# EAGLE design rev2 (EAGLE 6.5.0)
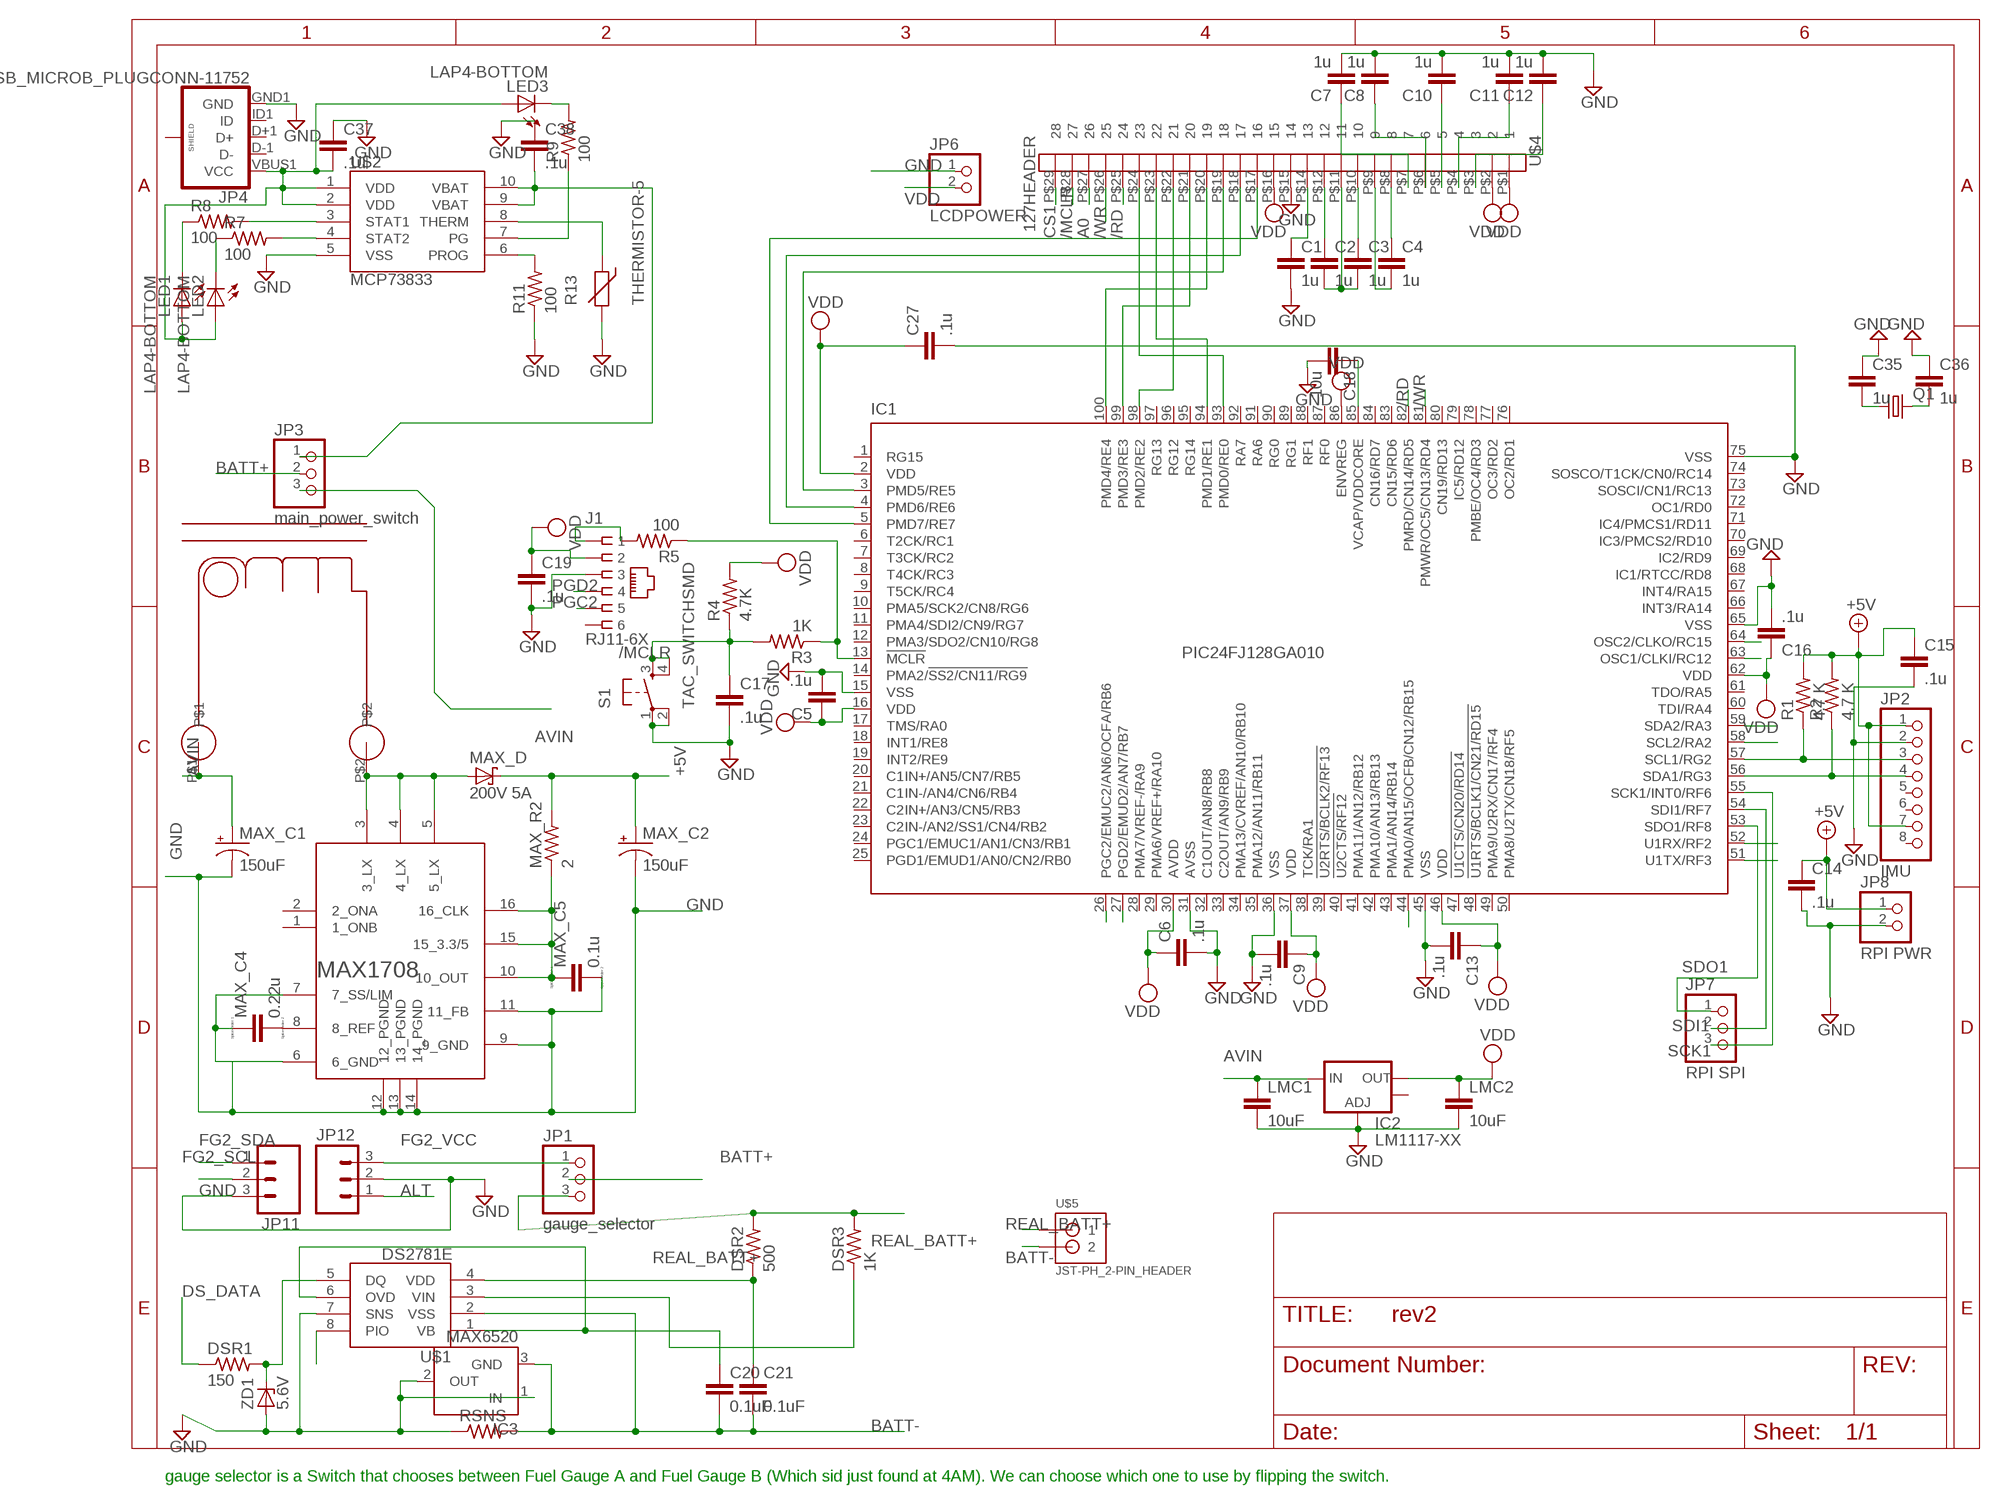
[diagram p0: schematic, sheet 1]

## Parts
C1  1u  C-EUC1206  [C1206]
C2  1u  C-EUC1206  [C1206]
C3  1u  C-EUC1206  [C1206]
C4  1u  C-EUC1206  [C1206]
C5  .1u  C-EUC1206  [C1206]
C6  .1u  C-EUC1206  [C1206]
C7  1u  C-EUC1206  [C1206]
C8  1u  C-EUC1206  [C1206]
C9  .1u  C-EUC1206  [C1206]
C10  1u  C-EUC1206  [C1206]
C11  1u  C-EUC1206  [C1206]
C12  1u  C-EUC1206  [C1206]
C13  .1u  C-EUC1206  [C1206]
C14  .1u  C-EUC1206  [C1206]
C15  .1u  C-EUC1206  [C1206]
C16  .1u  C-EUC1206  [C1206]
C17  .1u  C-EUC1206  [C1206]
C18  10u  C-EUC1206  [C1206]
C19  .1u  C-EUC1206  [C1206]
C20  0.1uF  C-EUC1206  [C1206]
C21  0.1uF  C-EUC1206  [C1206]
C27  .1u  C-EUC1206  [C1206]
C35  1u  C-EUC1206  [C1206]
C36  1u  C-EUC1206  [C1206]
C37  .1u  C-EUC1206  [C1206]
C38  .1u  C-EUC1206  [C1206]
DSR1  150  R-US_R1206  [R1206]
DSR2  500  R-US_R1206  [R1206]
DSR3  1K  R-US_R1206  [R1206]
IC1  PIC24FJ128GA010  [TQFP100-14X14]
IC2  LM1117-XX  V_REG_LM1117SOT223  [SOT223]
IC3  MAX6520  [SOT23]
J1  RJ11-6X  [RJ11-NO_SHIELD]
JP1  gauge_selector  PINHD-1X3  [1X03]
JP2  IMU  PINHD-1X8  [1X08]
JP3  main_power_switch  PINHD-1X3  [1X03]
JP4  USB_MICROB_PLUGCONN-11752  [USB-B-MICRO-SMD_V03]
JP6  LCDPOWER  PINHD-1X2  [1X02]
JP7  RPI SPI  PINHD-1X3  [1X03]
JP8  RPI PWR  PINHD-1X2  [1X02]
JP11  M03PTH  [1X03]
JP12  M03PTH  [1X03]
LED1  LAP4-BOTTOM  [P47F-BOTTOM]
LED2  LAP4-BOTTOM  [P47F-BOTTOM]
LED3  LAP4-BOTTOM  [P47F-BOTTOM]
LMC1  10uF  C-EUC1206  [C1206]
LMC2  10uF  C-EUC1206  [C1206]
MAX_C1  150uF  CPOL-USD/7343-31W  [D/7343-31W]
MAX_C2  150uF  CPOL-USD/7343-31W  [D/7343-31W]
MAX_C4  0.22u  CC1206  [C1206]
MAX_C5  0.1u  CC1206  [C1206]
MAX_D  200V 5A  SCHOTTKY-DIODESMC  [SMC]
MAX_R2  2  R-US_R1206  [R1206]
Q1  CRYTALHC49U-V  [HC49U-V]
R1  4.7 K  R-US_R1206  [R1206]
R2  4.7 K  R-US_R1206  [R1206]
R3  1K  R-US_R1206  [R1206]
R4  4.7K  R-US_R1206  [R1206]
R5  100  R-US_R1206  [R1206]
R7  100  R-US_R1206  [R1206]
R8  100  R-US_R1206  [R1206]
R9  100  R-US_R1206  [R1206]
R11  100  R-US_R1206  [R1206]
R13  THERMISTOR-5  [R-5]
RSNS  R-US_R1206  [R1206]
S1  TAC_SWITCHSMD  [TACTILE-SWITCH-SMD]
U$1  DS2781E  [TSSOP8]
U$2  MCP73833  [MSOP10]
U$3  MAX1708  [QSOP16]
U$4  127HEADER  [1.27HEADER]
U$5  JST-PH_2-PIN_HEADER  [JST_B2B-PH_HEADER]
U$6  UP2B-2R2-R  [UP2B-2R2-R]
ZD1  5.6V  ZENER-DIODESOD80C  [SOD80C]

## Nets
+5V: C14.1 C15.1 JP2.1 JP2.7 JP8.1 MAX_C2.+ MAX_D.C MAX_R2.2 R1.2 R2.2
/MCLR: C17.1 R3.2 R4.1 S1.3 S1.4 U$4.P$28
/RD: IC1.82(PMRD/CN14/RD5) U$4.P$25
/WR: IC1.81(PMWR/OC5/CN13/RD4) U$4.P$26
A0: IC1.44(PMA0/AN15/OCFB/CN12/RB15) U$4.P$27
ALT: JP12.1
AVIN: IC2.3(IN) JP3.3 LMC1.1 MAX_C1.+ U$6.P$1
BATT+: JP1.2 JP3.2
BATT-: C20.2 C21.2 IC3.3(GND) RSNS.2 U$1.2(VSS) U$5.P2
CS1: U$4.P$29
DS_DATA: DSR1.1 IC1.52(U1RX/RF2)
FG2_SCL: IC1.58(SCL2/RA2) JP11.2
FG2_SDA: IC1.59(SDA2/RA3) JP11.1
FG2_VCC: JP1.1 JP12.3
GND: C1.2 C5.2 C6.2 C7.2 C8.2 C9.2 C10.2 C11.2 C12.2 C13.2 C14.2 C15.2 C16.2 C17.2 C18.2 C19.2 C27.2 C35.1 C36.1 C37.1 C38.1 IC1.15(VSS) IC1.31(AVSS) IC1.36(VSS) IC1.45(VSS) IC1.65(VSS) IC1.75(VSS) IC2.1(ADJ) IC3.1(IN) IC3.2(OUT) J1.3 JP2.2 JP4.GND1(GND) JP6.1 JP8.2 JP11.3 JP12.2 LMC1.2 LMC2.2 MAX_C1.- MAX_C2.- MAX_C4.1 MAX_C5.2 R11.1 R13.2 RSNS.1 S1.1 S1.2 U$1.7(SNS) U$2.5(VSS) U$3.6(6_GND) U$3.7(7_SS/LIM) U$3.9(9_GND) U$3.11(11_FB) U$3.12(12_PGND) U$3.13(13_PGND) U$3.14(14_PGND) U$4.P$15 ZD1.A
N$1: IC1.57(SCL1/RG2) JP2.3 R1.1
N$2: IC1.56(SDA1/RG3) JP2.4 R2.1
N$3: LED1.C R8.1
N$4: IC1.13(!MCLR) R3.1 R5.1
N$5: R8.2 U$2.3(STAT1)
N$6: R7.2 U$2.4(STAT2)
N$7: C18.1 IC1.85(VCAP/VDDCORE)
N$8: IC1.5(PMD7/RE7) U$4.P$17
N$9: IC1.4(PMD6/RE6) U$4.P$18
N$10: IC1.3(PMD5/RE5) U$4.P$19
N$11: IC1.100(PMD4/RE4) U$4.P$20
N$12: IC1.99(PMD3/RE3) U$4.P$21
N$13: IC1.98(PMD2/RE2) U$4.P$22
N$14: IC1.94(PMD1/RE1) U$4.P$23
N$15: IC1.93(PMD0/RE0) U$4.P$24
N$16: C7.1 U$4.P$7
N$17: C3.1 U$4.P$10
N$18: LED2.C R7.1
N$19: C2.1 U$4.P$12
N$20: C2.2 C3.2 U$4.P$11
N$21: C1.1 U$4.P$14
N$22: C4.2 U$4.P$9
N$23: C4.1 U$4.P$8
N$24: C8.1 U$4.P$6
N$25: C10.1 U$4.P$5
N$26: C11.1 U$4.P$4
N$27: C12.1 U$4.P$3
N$28: R9.1 U$2.7(PG)
N$29: J1.1 R5.2
N$31: DSR1.2 U$1.5(DQ) ZD1.C
N$32: LED3.C R9.2
N$33: R11.2 U$2.6(PROG)
N$34: R13.1 U$2.8(THERM)
N$35: MAX_D.A U$3.3(3_LX) U$3.4(4_LX) U$3.5(5_LX) U$6.P$2
N$36: C21.1 DSR2.1 U$1.4(VDD)
N$37: C20.1 U$1.1(VB) U$1.6(OVD)
N$38: MAX_C5.1 MAX_R2.1 U$3.10(10_OUT) U$3.15(15_3.3/5) U$3.16(16_CLK)
N$39: DSR3.1 U$1.3(VIN)
N$40: MAX_C4.2 U$3.8(8_REF)
N$51: C38.2 JP3.1 U$2.9(VBAT) U$2.10(VBAT)
OSC1: C36.2 IC1.63(OSC1/CLKI/RC12) Q1.2
OSC2: C35.2 IC1.64(OSC2/CLKO/RC15) Q1.1
PGC2: IC1.26(PGC2/EMUC2/AN6/OCFA/RB6) J1.5
PGD2: IC1.27(PGD2/EMUD2/AN7/RB7) J1.4
PIO: IC1.51(U1TX/RF3) U$1.8(PIO)
REAL_BATT+: DSR2.2 DSR3.2 JP1.3 U$5.P1
SCK1: IC1.55(SCK1/INT0/RF6) JP7.3
SDI1: IC1.54(SDI1/RF7) JP7.2
SDO1: IC1.53(SDO1/RF8) JP7.1
VDD: C5.1 C6.1 C9.1 C13.1 C16.1 C19.1 C27.1 IC1.2(VDD) IC1.16(VDD) IC1.30(AVDD) IC1.37(VDD) IC1.46(VDD) IC1.62(VDD) IC1.86(ENVREG) IC2.2(OUT) J1.2 JP6.2 LMC2.1 R4.2 U$4.P$1 U$4.P$2 U$4.P$16
VDDUSB: C37.2 JP4.VBUS1(VCC) LED1.A LED2.A LED3.A U$2.1(VDD) U$2.2(VDD)
Unconnected: IC1.1(RG15) IC1.6(T2CK/RC1) IC1.7(T3CK/RC2) IC1.8(T4CK/RC3) IC1.9(T5CK/RC4) IC1.10(PMA5/SCK2/CN8/RG6) IC1.11(PMA4/SDI2/CN9/RG7) IC1.12(PMA3/SDO2/CN10/RG8) IC1.14(PMA2/!SS2/CN11/RG9) IC1.17(TMS/RA0) IC1.18(INT1/RE8) IC1.19(INT2/RE9) IC1.20(C1IN+/AN5/CN7/RB5) IC1.21(C1IN-/AN4/CN6/RB4) IC1.22(C2IN+/AN3/CN5/RB3) IC1.23(C2IN-/AN2/SS1/CN4/RB2) IC1.24(PGC1/EMUC1/AN1/CN3/RB1) IC1.25(PGD1/EMUD1/AN0/CN2/RB0) IC1.28(PMA7/VREF-/RA9) IC1.29(PMA6/VREF+/RA10) IC1.32(C1OUT/AN8/RB8) IC1.33(C2OUT/AN9/RB9) IC1.34(PMA13/CVREF/AN10/RB10) IC1.35(PMA12/AN11/RB11) IC1.38(TCK/RA1) IC1.39(!U2RTS/BCLK2/RF13) IC1.40(!U2CTS/RF12) IC1.41(PMA11/AN12/RB12) IC1.42(PMA10/AN13/RB13) IC1.43(PMA1/AN14/RB14) IC1.47(!U1CTS/CN20/RD14) IC1.48(!U1RTS/BCLK1/CN21/RD15) IC1.49(PMA9/U2RX/CN17/RF4) IC1.50(PMA8/U2TX/CN18/RF5) IC1.60(TDI/RA4) IC1.61(TDO/RA5) IC1.66(INT3/RA14) IC1.67(INT4/RA15) IC1.68(IC1/RTCC/RD8) IC1.69(IC2/RD9) IC1.70(IC3/PMCS2/RD10) IC1.71(IC4/PMCS1/RD11) IC1.72(OC1/RD0) IC1.73(SOSCI/CN1/RC13) IC1.74(SOSCO/T1CK/CN0/RC14) IC1.76(OC2/RD1) IC1.77(OC3/RD2) IC1.78(PMBE/OC4/RD3) IC1.79(IC5/RD12) IC1.80(CN19/RD13) IC1.83(CN15/RD6) IC1.84(CN16/RD7) IC1.87(RF0) IC1.88(RF1) IC1.89(RG1) IC1.90(RG0) IC1.91(RA6) IC1.92(RA7) IC1.95(RG14) IC1.96(RG12) IC1.97(RG13) IC2.4(OUT) J1.6 JP2.5 JP2.6 JP2.8 JP4.D+1(D+) JP4.D-1(D-) JP4.ID1(ID) JP4.SHIELD1(SHIELD) JP4.SHIELD2(SHIELD) JP4.SHIELD3(SHIELD) U$3.1(1_ONB) U$3.2(2_ONA)

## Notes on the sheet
- gauge selector is a Switch that chooses between Fuel Gauge A and Fuel Gauge B (Which sid just found at 4AM). We can choose which one to use by flipping the switch.

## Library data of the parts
C1-C21 C27 C35-C38 LMC1 LMC2 = rcl:C-EU: CAPACITOR, European symbol
DSR1-DSR3 R1-R5 R7-R9 R11 RSNS = rcl:R-US_: RESISTOR, American symbol
IC1 = microchip:PIC24FJ*GA010: 64/80/100-Pin General Purpose, 16-Bit Flash Microcontrollers Source: http://ww1.microchip.com/downloads/en/DeviceDoc/39747d.pdf; MPN: PIC24FJ128GA010-I/PT; OC_FARNELL: 1146522; OC_NEWARK: 56K7341
IC2 = SparkFun-PowerIC:V_REG_LM1117: Voltage Regulator LM1117 Standard adjustable voltage regulator but in SMD form. Spark Fun Electronics SKU : COM-00595; PROD_ID: VREG-08170
IC3 = maxim:MAX6520: 1.2V Voltage Reference 50ppm/°C, SOT23, 3-Terminal Source: Data sheet; MF: MAXIM; MPN: MAX6520EUR-T; OC_FARNELL: unknown; OC_NEWARK: 02J4586
J1 = con-tycoelectronics:RJ11: CORCOM Modular RJ Jacks No Shield Source: www.tycoelectronics.com .. ENG_DS_1654001_1099_RJ_L_0507.pdf; MPN: RJ11-6X; OC_FARNELL: unknown; OC_NEWARK: 16R6089
JP1 JP3 JP7 = pinhead:PINHD-1X3: PIN HEADER
JP2 = pinhead:PINHD-1X8: PIN HEADER
JP4 = SparkFun-Connectors:USB_MICROB_PLUG: USB Micro-B connectors Some male, some female. Watch your step!
JP6 JP8 = pinhead:PINHD-1X2: PIN HEADER
JP11 JP12 = SparkFun:M03: Header 3 Standard 3-pin 0.1" header. Use with straight break away headers (SKU : PRT-00116), right angle break away headers (PRT-00553), swiss pins (PRT-00743), machine pins (PRT-00117), and female headers (PRT-00115). Molex polarized connector foot print use with SKU : PRT-08232 with associated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
LED1-LED3 = led:*P4: PointLED® Enhanced Thinfilm LED TOP & BOTTOM mount
MAX_C1 MAX_C2 = adafruit:CPOL-US: POLARIZED CAPACITOR, American symbol
MAX_C4 MAX_C5 = eagle-ltspice:C: CAPACITOR, European symbol; SPICEMODEL: NONE; SPICEPREFIX: C
MAX_D = diode:SCHOTTKY-DIODE: Schottky Diode
MAX_R2 = adafruit:R-US_: RESISTOR, American symbol
Q1 = crystal:CRYTAL: CRYSTAL
R13 = varistor:THERMISTOR: THERMISTOR
S1 = SparkFun-Retired:TAC_SWITCH: Momentary Switch Button commonly used for reset or general input. Spark Fun Electronics SKU : COM-00097 SMT- SWCH-08247; PROD_ID: SWCH-08247
U$1 = fuelgauge:DS2781E
U$2 = fuelgauge:MCP73833
U$3 = max1708:MAX1708
U$4 = fuelgauge:127HEADER
U$5 = SRG:JST-PH_2-PIN_HEADER: 2-pin JST PH Shrouded Header, top entry
U$6 = duckgauge:UP2B-2R2-R: Yeah yeah inducktor
ZD1 = diode:ZENER-DIODE: Z-Diode

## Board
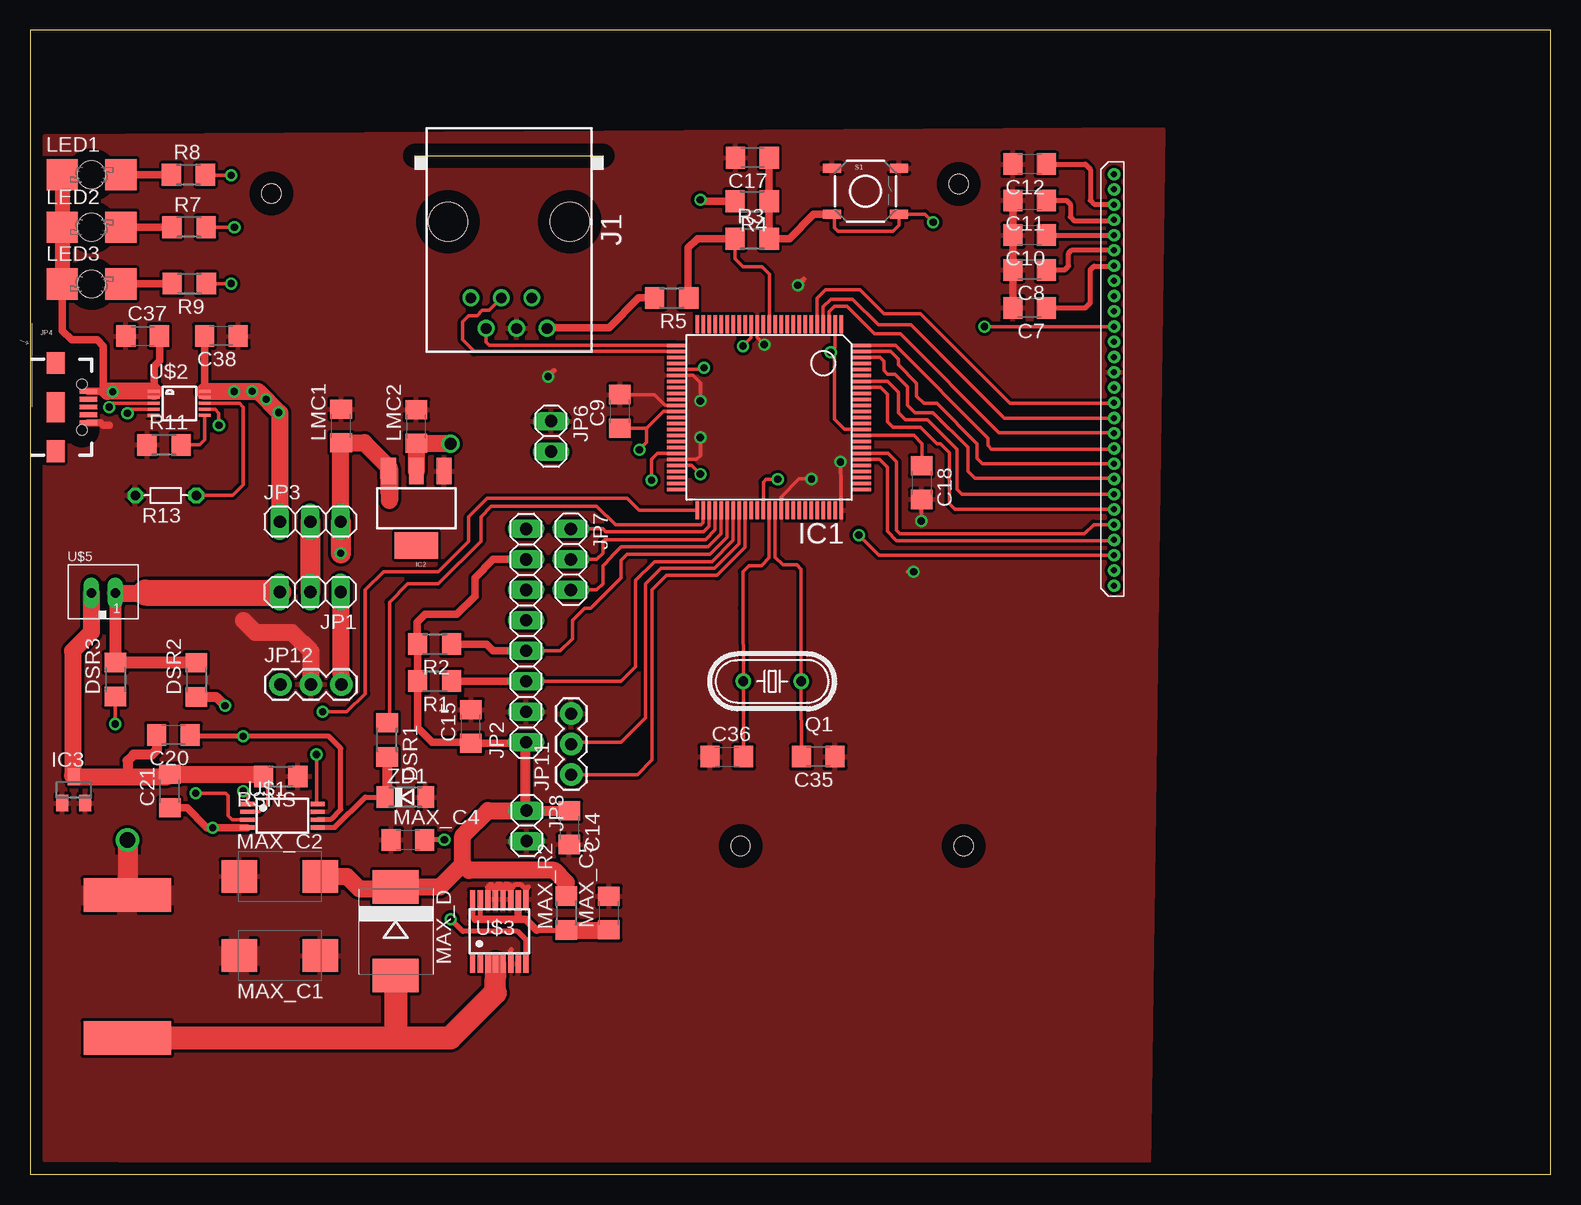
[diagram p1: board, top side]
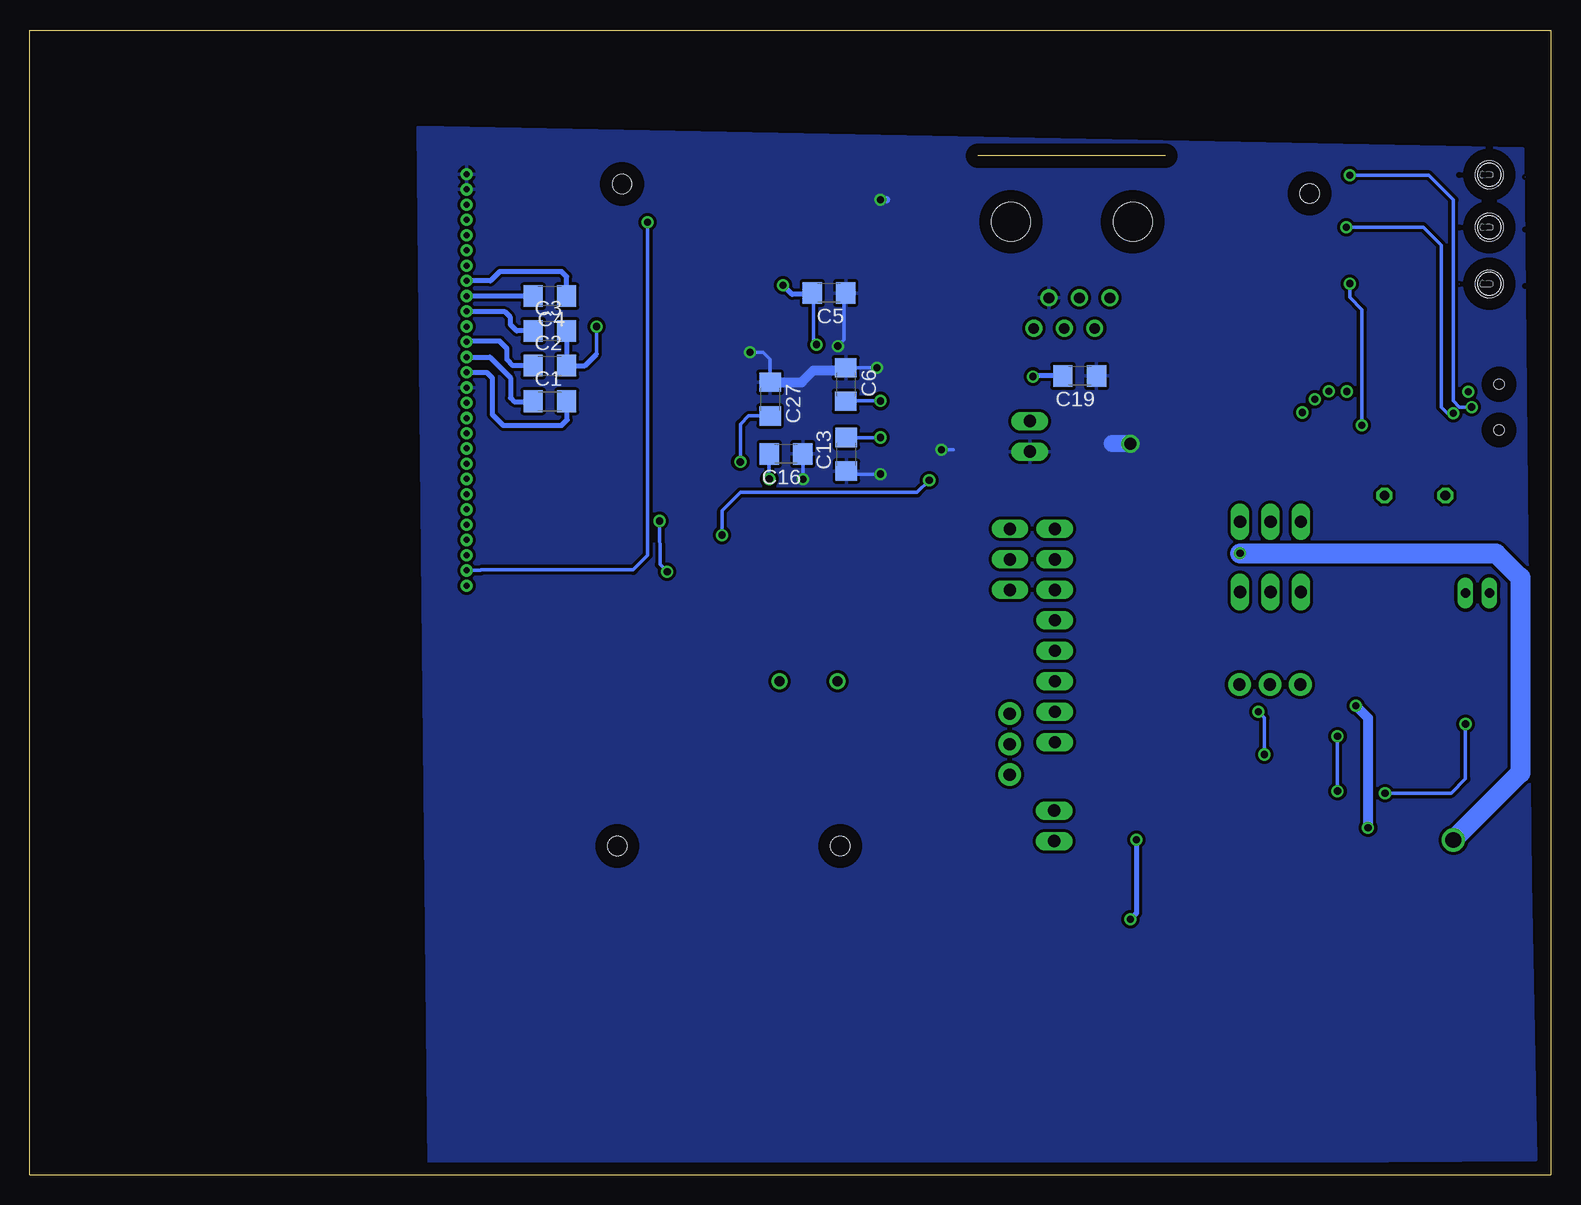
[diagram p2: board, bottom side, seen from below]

Size 126.78 x 95.4 mm. Coordinates in mm from the lower left corner, seen from the top.
Outline: 126.78,0 126.78,95.4 0,95.4 0,0 126.78,0
Copper layers (1*16): Top 0.035mm / dielectric 1.5mm / Bottom 0.035mm
Design rules "default": minimum track width 10mil, minimum drill 24mil, track to track 8mil, track to pad 8mil, pad to pad 8mil, via to via 8mil, smd to smd 8mil, copper to edge 40mil, drill to drill 8mil, minimum pad ring 10mil, minimum via ring 8mil, stop-mask expansion 4mil, vias tented up to drill 0mil, thermal gap 10mil
Holes 1.6 mm at 59.23,27.41 77.42,82.58 20.12,81.76 77.83,27.41

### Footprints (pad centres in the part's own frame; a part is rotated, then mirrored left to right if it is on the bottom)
C1206 = smd 1.6 x 1.8: 1 -1.4,0; 2 1.4,0
R1206 = smd 1.6 x 1.803: 1 -1.422,0; 2 1.422,0
TQFP100-14X14 = smd 0.27 x 1.5: 1 -6,-7.75; 2 -5.5,-7.75; 3 -5,-7.75; 4 -4.5,-7.75; 5 -4,-7.75; 6 -3.5,-7.75; 7 -3,-7.75; 8 -2.5,-7.75; 9 -2,-7.75; 10 -1.5,-7.75; 11 -1,-7.75; 12 -0.5,-7.75; 13 0,-7.75; 14 0.5,-7.75; 15 1,-7.75; 16 1.5,-7.75; 17 2,-7.75; 18 2.5,-7.75; 19 3,-7.75; 20 3.5,-7.75; 21 4,-7.75; 22 4.5,-7.75; 23 5,-7.75; 24 5.5,-7.75; 25 6,-7.75; 51 6,7.75; 52 5.5,7.75; 53 5,7.75; 54 4.5,7.75; 55 4,7.75; 56 3.5,7.75; 57 3,7.75; 58 2.5,7.75; 59 2,7.75; 60 1.5,7.75; 61 1,7.75; 62 0.5,7.75; 63 0,7.75; 64 -0.5,7.75; 65 -1,7.75; 66 -1.5,7.75; 67 -2,7.75; 68 -2.5,7.75; 69 -3,7.75; 70 -3.5,7.75; 71 -4,7.75; 72 -4.5,7.75; 73 -5,7.75; 74 -5.5,7.75; 75 -6,7.75 | smd 1.5 x 0.27: 26 7.75,-6; 27 7.75,-5.5; 28 7.75,-5; 29 7.75,-4.5; 30 7.75,-4; 31 7.75,-3.5; 32 7.75,-3; 33 7.75,-2.5; 34 7.75,-2; 35 7.75,-1.5; 36 7.75,-1; 37 7.75,-0.5; 38 7.75,0; 39 7.75,0.5; 40 7.75,1; 41 7.75,1.5; 42 7.75,2; 43 7.75,2.5; 44 7.75,3; 45 7.75,3.5; 46 7.75,4; 47 7.75,4.5; 48 7.75,5; 49 7.75,5.5; 50 7.75,6; 76 -7.75,6; 77 -7.75,5.5; 78 -7.75,5; 79 -7.75,4.5; 80 -7.75,4; 81 -7.75,3.5; 82 -7.75,3; 83 -7.75,2.5; 84 -7.75,2; 85 -7.75,1.5; 86 -7.75,1; 87 -7.75,0.5; 88 -7.75,0; 89 -7.75,-0.5; 90 -7.75,-1; 91 -7.75,-1.5; 92 -7.75,-2; 93 -7.75,-2.5; 94 -7.75,-3; 95 -7.75,-3.5; 96 -7.75,-4; 97 -7.75,-4.5; 98 -7.75,-5; 99 -7.75,-5.5; 100 -7.75,-6
SOT223 = smd 1.219 x 2.235: 1 -2.311,-3.099; 2 0,-3.099; 3 2.311,-3.099 | smd 3.6 x 2.2: 4 0,3.099
SOT23 = smd 1 x 1.4: 1 -0.95,-1.1; 2 0.95,-1.1; 3 0,1.1
RJ11-NO_SHIELD = drill 0.9 pad 1.4: 1 -3.175,8.89; 2 -1.905,6.35; 3 -0.635,8.89; 4 0.635,6.35; 5 1.905,8.89; 6 3.175,6.35 | hole 3.251: -5.08,0; 5.08,0
1X03 = drill 1.016 long: 1 -2.54,0; 2 0,0; 3 2.54,0
1X08 = drill 1.016 long: 1 -8.89,0; 2 -6.35,0; 3 -3.81,0; 4 -1.27,0; 5 1.27,0; 6 3.81,0; 7 6.35,0; 8 8.89,0
USB-B-MICRO-SMD_V03 = smd 1.45 x 0.4: D+1 2.725,0; D-1 2.725,0.65; GND1 2.725,-1.3; ID1 2.725,-0.65; VBUS1 2.725,1.3 | smd 1.5 x 1.8: SHIELD1 0,3.685; SHIELD2 0,-3.685 | smd 1.5 x 2.5: SHIELD3 0,0 | hole 0.85: 2.2,1.9; 2.2,-1.9
1X02 = drill 1.016 long: 1 -1.27,0; 2 1.27,0
1X03' = drill 1.016 pad 1.88: 1 0,0; 2 2.54,0; 3 5.08,0
P47F-BOTTOM = smd 2.6 x 2.6: A -2.45,0; C 2.45,0 | hole 2.3: 0,0
D/7343-31W = smd 2.95 x 2.7: + 3.375,0; - -3.375,0
SMC = smd 2.8 x 3.8: A 3.7,0; C -3.7,0
HC49U-V = drill 0.813: 1 -2.413,0; 2 2.413,0
R-5 = drill 0.813 octagon: 1 -2.54,0; 2 2.54,0
TACTILE-SWITCH-SMD = smd 1.524 x 0.762: 1 -2.794,1.905; 2 2.794,1.905; 3 -2.794,-1.905; 4 2.794,-1.905
TSSOP8 = smd 1.2 x 0.35: 1 -2.925,0.975; 2 -2.925,0.325; 3 -2.925,-0.325; 4 -2.925,-0.975; 5 2.925,-0.975; 6 2.925,-0.325; 7 2.925,0.325; 8 2.925,0.975
MSOP10 = smd 0.25 x 1: 1 -1,-2.113; 2 -0.5,-2.113; 3 0,-2.113; 4 0.5,-2.113; 5 1,-2.113; 6 1,2.113; 7 0.5,2.113; 8 0,2.113; 9 -0.5,2.113; 10 -1,2.113
QSOP16 = smd 0.45 x 1.5: 1 -2.223,-2.69; 2 -1.587,-2.69; 3 -0.953,-2.69; 4 -0.318,-2.69; 5 0.318,-2.69; 6 0.953,-2.69; 7 1.587,-2.69; 8 2.223,-2.69; 9 2.223,2.69; 10 1.587,2.69; 11 0.953,2.69; 12 0.318,2.69; 13 -0.318,2.69; 14 -0.953,2.69; 15 -1.587,2.69; 16 -2.223,2.69
1.27HEADER = drill 0.5 pad 1.016: P$1 0.406,0.457; P$2 1.676,0.457; P$3 2.946,0.457; P$4 4.216,0.457; P$5 5.486,0.457; P$6 6.756,0.457; P$7 8.026,0.457; P$8 9.296,0.457; P$9 10.566,0.457; P$10 11.836,0.457; P$11 13.106,0.457; P$12 14.376,0.457; P$14 15.646,0.457; P$15 16.916,0.457; P$16 18.186,0.457; P$17 19.456,0.457; P$18 20.726,0.457; P$19 21.996,0.457; P$20 23.266,0.457; P$21 24.536,0.457; P$22 25.806,0.457; P$23 27.076,0.457; P$24 28.346,0.457; P$25 29.616,0.457; P$26 30.886,0.457; P$27 32.156,0.457; P$28 33.426,0.457; P$29 34.696,0.457
JST_B2B-PH_HEADER = drill 0.8 long: P1 1.075,0.048; P2 -0.925,0.048
UP2B-2R2-R = smd 2.8 x 7.3: P$1 -19.27,1; P$2 -7.365,1
SOD80C = smd 1.4 x 1.8: A 1.7,0; C -1.7,0

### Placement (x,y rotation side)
C1  83.44,64.47 0 bottom
C2  83.44,67.44 0 bottom
C3  83.44,70.33 0 bottom
C4  83.44,73.23 180 bottom
C5  60.17,73.48 180 bottom
C6  58.78,65.86 270 bottom
C7  83.34,72.24 180 top
C8  83.34,75.41 180 top
C9  49.17,63.63 90 top
C10  83.34,78.31 180 top
C11  83.34,81.2 180 top
C12  83.34,84.23 180 top
C13  58.72,60.05 90 bottom
C14  44.96,28.93 270 top
C15  36.75,37.36 90 top
C16  63.75,60.07 180 bottom
C17  60.22,84.76 180 top
C18  74.32,57.68 270 top
C19  39.27,66.57 180 bottom
C20  11.96,36.65 180 top
C21  11.66,31.98 90 top
C27  65.07,64.64 270 bottom
C35  65.71,34.85 180 top
C36  58.09,34.85 0 top
C37  9.4,69.9 0 top
C38  15.95,69.9 180 top
DSR1  29.77,36.25 270 top
DSR2  13.87,41.25 90 top
DSR3  7.11,41.27 90 top
IC1  61.62,63.12 180 top
IC2  32.21,55.55 180 top
IC3  3.66,32.08 0 top
J1  39.93,79.43 180 top
JP1  23.37,48.56 180 top
JP2  41.35,44.93 90 top
JP3  23.37,54.43 0 top
JP4  2.13,63.98 0 top
JP6  43.43,61.54 270 top
JP7  45.09,51.28 270 top
JP8  41.4,29.08 270 top
JP11  [1X03']  45.11,33.35 90 top
JP12  [1X03']  20.88,40.87 0 top
LED1  5.13,83.34 0 top
LED2  5.13,78.97 0 top
LED3  5.13,74.24 0 top
LMC1  25.93,62.41 90 top
LMC2  32.21,62.36 90 top
MAX_C1  20.83,18.26 180 top
MAX_C2  20.83,24.87 0 top
MAX_C4  31.5,27.91 0 top
MAX_C5  48.26,21.82 90 top
MAX_D  30.48,20.29 270 top
MAX_R2  44.7,21.82 90 top
Q1  61.87,41.12 180 top
R1  33.73,41.15 180 top
R2  33.73,44.22 180 top
R3  60.2,78 0 top
R4  60.2,81.13 180 top
R5  53.49,73.08 180 top
R7  13.26,78.97 0 top
R8  13.21,83.34 0 top
R9  13.28,74.27 180 top
R11  11.18,60.83 0 top
R13  11.33,56.62 180 top
RSNS  20.9,33.2 180 top
S1  69.65,81.97 0 top
U$1  21.06,29.92 0 top
U$2  12.45,64.29 270 top
U$3  39.12,20.29 0 top
U$4  89.92,83.79 270 top
U$5  6.05,48.44 0 top
U$6  7.11,4.04 270 top
ZD1  31.29,31.47 0 top

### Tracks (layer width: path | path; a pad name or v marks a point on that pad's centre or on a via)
+5V
  Top 0.61: JP2.7 38.61,51.28 37.08,49.76 37.08,48.23 35.56,46.71 32.94,46.71 32.28,46.05 32.28,44.25 R2.2 R1.2 32.31,37.26 33.53,36.04 36.67,36.04 C15.1 41.27,35.96 JP2.1
  Top 0.813: 41.27,35.96 41.27,30.48 JP8.1 44.94,30.35 C14.1
  Top 1.422: MAX_C2.+ 26.42,24.87 27.43,23.85 30.34,23.85 MAX_D.C 34.18,23.99 36.07,25.88 | 36.07,25.88 36.07,28.24 38.18,30.35 JP8.1 | MAX_R2.2 44.7,24.36 43.69,25.37 36.58,25.37 36.07,25.88
/MCLR  (via drill 0.6)
  Top 0.305: S1.3 67.06,79.86 67.06,78.92 67.36,78.61 71.93,78.61 72.44,79.12 S1.4 74.6,80.06 v75.29,79.37
  Top 0.61: S1.3 66.83,80.04 65.33,80.04 63.3,78 R3.2 R4.1 C17.1
  Bottom 0.305: v75.29,79.37 75.29,51.64 76.5,50.42 89.15,50.42 89.2,50.37 U$4.P$28
/RD
  Top 0.305: IC1.82 71.53,60.12 72.24,59.41 72.24,53.7 72.52,53.42 87.91,53.42 88.67,54.18 U$4.P$25
/WR
  Top 0.305: IC1.81 70.81,59.62 71.48,58.95 71.48,53.62 72.24,52.86 90.32,52.86 U$4.P$26
A0  (via drill 0.6)
  Top 0.305: U$4.P$27 70.76,51.64 v69.09,53.31 | v51.82,57.89 51.82,59.64 52.32,60.15 53.84,60.15 IC1.44
  Bottom 0.305: v69.09,53.31 69.09,55.35 67.56,56.87 52.83,56.87 v51.82,57.89
AVIN  (via drill 0.6, 1.3)
  Top 1.422: IC2.3 29.97,56.18 29.97,58.9 27.87,61.01 LMC1.1 25.91,60.98 JP3.3
  Top 1.676: JP3.3 v25.91,51.79 | v8.13,27.91 8.13,23.32 U$6.P$1
  Bottom 1.676: v25.91,51.79 4.57,51.79 2.54,49.76 2.54,33.5 v8.13,27.91
  pour Top: 3.05,25.88 10.67,25.88 12.19,24.36 12.19,21.31 13.21,20.29 19.3,20.29 19.81,19.79 19.81,17.25 18.8,16.23 4.06,16.23 3.05,17.25
BATT+
  Top 1.676: JP3.2 JP1.2
BATT-
  Top 0.305: U$1.2 19.12,30.25 19.12,30.27 19.81,30.96 19.81,32.87 RSNS.2 19.56,33.12
  Top 0.813: C20.2 10.56,35.43 10.16,35.03 8.64,35.03 8.13,34.52 8.13,33.18
  Top 1.422: U$5.P2 5.12,45.23 3.56,43.66 3.56,33.28 IC3.3 8.13,33.18 11.46,33.18 C21.2 | 11.6,33.32 C21.2 | C21.2 19.3,33.38 RSNS.2
DS_DATA
  Top 0.305: IC1.52 56.12,54.34 55.93,54.15 48.79,54.15 47.24,55.7 38.46,55.7 37.59,54.84 37.59,52.81 34.04,49.25 31.5,49.25 29.97,47.73 29.97,37.87 DSR1.1
FG2_SCL
  Top 0.305: IC1.58 59.12,52.59 57.07,50.55 52.6,50.55 51.31,49.25 51.31,38.07 49.28,36.04 45.26,36.04 JP11.2
FG2_SDA
  Top 0.305: IC1.59 59.62,52.31 57.28,49.96 53.06,49.96 51.87,48.77 51.87,34.57 50.65,33.35 JP11.1
FG2_VCC
  Top 1.422: JP1.1 25.91,41.94 JP12.3
GND  (via drill 0.6)
  Top 0.305: IC1.36 52.95,64.12 52.05,65.02 50.7,65.02 C9.2 | IC1.15 60.62,69.78 v61.21,69.19 | IC1.31 55.28,66.62 55.88,66.01 v55.88,64.49 | IC1.45 55.58,59.62 55.88,59.92 v55.88,61.44 | IC1.75 67.62,57.32 v67.56,59.41 | v65.15,57.99 64.11,57.99 62.64,56.51 62.64,55.35 | 62.64,54.79 62.64,55.35 | 62.64,55.35 IC1.65 | C18.2 74.32,54.74 v74.3,54.48 | v73.66,50.27 73.15,50.27
  Top 0.406: v64.01,74.14 64.52,74.65 | v43.18,66.52 43.69,67.03 | U$3.6 40.07,18.71 40.13,18.77 | U$3.11 40.07,24.09 40.03,24.13 39.98,24.13 39.9,24.21 39.57,24.21 39.42,24.05 | 39.42,23.39 39.42,24.05 | 39.42,24.05 39.24,24.23 38.96,24.23 38.76,24.03 38.76,23.27 38.81,23.22 38.81,23.85 38.48,24.18 38.35,24.18 38.12,23.95 38.12,23.34 38.2,23.27 38.2,23.98 38.23,24 38.35,24 38.46,24.1 38.46,23.95 38.51,23.9 40.16,23.9 40.18,23.88 40.18,23.9 40.49,24.21 40.89,24.21 41.12,23.98 41.5,23.98 | 41.53,23.98 41.5,23.98 | 41.5,23.98 41.3,23.77 41.3,23.02 U$3.9
  Top 0.61: C11.2 C10.2 C8.2 C7.2 | JP4.GND1 5.87,62.68 6.1,62.46 6.6,62.46
  Top 1.422: JP12.2 23.42,43.61 21.84,45.19 18.8,45.19 17.78,46.2
  Bottom 0.305: v61.21,69.19 61.21,69.32 61.47,69.57 61.47,73.38 C5.2 | v55.88,64.49 58.75,64.49 C6.2 | v55.88,61.44 C13.2 | v67.56,59.41 67.56,62.56 66.88,63.25 C27.2 | C16.2 v65.15,57.99 | v74.3,54.48 74.27,50.88 v73.66,50.27
  Bottom 0.406: U$4.P$15 88.7,66.88 88.24,66.42 88.24,63.37 87.33,62.46 82.45,62.46 81.99,62.92 81.99,64.42 C1.2 | 61.47,73.38 63.24,73.38 v64.01,74.14 | C19.2 43.13,66.57 v43.18,66.52
  pour Top (isolate 0.254): 1.27,86.54 94.44,87.15 93.22,0.63 1.27,1.24
N$1
  Top 0.305: IC1.57 58.62,52.88 56.84,51.1 52.05,51.1 50.49,49.56 50.49,42.34 49.28,41.12 JP2.3
  Top 0.61: R1.1 41.33,41.15 JP2.3
N$2
  Top 0.305: IC1.56 58.12,53.14 56.69,51.71 49.78,51.71 49.28,51.21 49.28,49.76 46.74,47.22 46.23,47.22 45.21,46.2 45.21,44.68 44.2,43.66 JP2.4
  Top 0.61: R2.1 38.05,44.22 38.61,43.66 JP2.4
N$3
  Top 0.61: LED1.C R8.1
N$4
  Top 0.305: R3.1 58.78,76.33 59.44,75.67 61.01,75.67 61.65,75.03 61.65,70.89 IC1.13
  Top 0.61: R3.1 55.63,78 54.86,77.24 54.86,73.13 R5.1
N$5  (via drill 0.6)
  Top 0.305: U$2.3 6.91,64.29 v6.6,63.98 | v16.76,83.29 14.68,83.29 R8.2
  Bottom 0.305: v16.76,83.29 10.16,83.29 8.13,81.25 8.13,64.49 7.62,63.98 v6.6,63.98
N$6  (via drill 0.6)
  Top 0.305: U$2.4 8.44,63.79 v8.13,63.47 | v17.04,78.97 R7.2
  Bottom 0.305: v17.04,78.97 10.64,78.97 9.14,77.47 9.14,63.98 8.64,63.47 v8.13,63.47
N$7
  Top 0.305: IC1.85 73.69,61.62 74.37,60.93 74.37,59.13 C18.1
N$8
  Top 0.305: IC1.5 65.62,73.06 66.29,73.74 69.19,73.74 71.17,71.75 74.22,71.75 81.69,64.29 90.32,64.29 U$4.P$17
N$9
  Top 0.305: IC1.4 66.12,72.34 66.75,72.97 68.58,72.97 70.71,70.84 73.46,70.84 81.23,63.07 U$4.P$18
N$10
  Top 0.305: IC1.3 66.62,71.93 67.06,72.36 68.12,72.36 70.41,70.08 72.54,70.08 80.77,61.85 90.32,61.85 U$4.P$19
N$11
  Top 0.305: IC1.100 72.13,69.12 79.86,61.39 79.86,60.78 80.16,60.48 90.32,60.48 U$4.P$20
N$12
  Top 0.305: IC1.99 71.72,68.62 72.39,67.94 72.39,67.49 73.91,65.96 73.91,64.9 74.52,64.29 75.59,64.29 78.94,60.93 78.94,59.72 79.4,59.26 U$4.P$21
N$13
  Top 0.305: IC1.98 70.84,68.12 71.17,67.79 71.17,67.03 71.48,66.73 72.08,66.73 73.15,65.66 73.15,64.13 73.76,63.53 75.29,63.53 78.18,60.63 78.18,58.65 78.79,58.04 90.32,58.04 U$4.P$22
N$14
  Top 0.305: U$4.P$23 77.67,56.72 77.27,57.12 77.27,60.48 74.83,62.92 73,62.92 72.39,63.53 72.39,65.2 71.48,66.12 IC1.94
N$15
  Top 0.305: IC1.93 70.91,65.62 71.48,65.05 71.48,62.76 71.93,62.31 74.22,62.31 75.59,60.93 75.89,60.93 76.66,60.17 76.66,55.91 77.11,55.45 U$4.P$24
N$16
  Top 0.406: C7.1 87.96,72.24 88.39,72.67 88.39,75.41 88.7,75.72 90.32,75.72 U$4.P$7
N$17
  Bottom 0.406: C3.1 86.21,70.33 86.72,70.84 86.72,71.45 87.17,71.91 90.32,71.91 U$4.P$10
N$18
  Top 0.61: LED2.C R7.1
N$19
  Bottom 0.406: C2.1 86.51,67.44 87.02,67.94 87.02,68.86 87.63,69.47 90.32,69.47 U$4.P$12
N$20  (via drill 0.6)
  Top 0.305: U$4.P$11 v79.55,70.69
  Bottom 0.305: v79.55,70.69 79.55,68.4
  Bottom 0.406: C3.2 C2.2 80.52,67.44 79.55,68.4
N$21
  Bottom 0.406: U$4.P$14 88.44,68.15 86.72,66.42 86.72,64.74 86.41,64.44 84.86,64.44 C1.1
N$22
  Bottom 0.406: C4.2 U$4.P$9
N$23
  Bottom 0.406: C4.1 82.04,74.85 82.45,75.26 87.63,75.26 88.39,74.5 U$4.P$8
N$24
  Top 0.406: C8.1 86.26,75.41 86.56,75.72 86.56,76.78 86.87,77.09 90.32,77.09 U$4.P$6
N$25
  Top 0.406: C10.1 U$4.P$5
N$26
  Top 0.406: C11.1 86.41,81.2 86.72,80.9 86.72,79.83 87.02,79.53 90.32,79.53 U$4.P$4
N$27
  Top 0.406: C12.1 87.96,84.23 88.39,83.79 88.39,81.2 88.7,80.9 90.32,80.9 U$4.P$3
N$28  (via drill 0.6)
  Top 0.305: U$2.7 15.44,63.79 15.75,63.47 v15.75,62.46 | v16.76,74.27 R9.1
  Bottom 0.305: v15.75,62.46 15.75,72.11 16.76,73.13 v16.76,74.27
N$29
  Top 0.61: J1.1 43.16,70.59 48.26,70.59 50.75,73.08 R5.2
N$31
  Top 0.406: U$1.5 25.42,28.95 27.94,31.47 ZD1.C
  Top 0.813: DSR1.2 29.77,31.65 ZD1.C
N$32
  Top 0.61: LED3.C 11.28,74.24 R9.2
N$33
  Top 0.305: U$2.6 14.56,61.24 14.15,60.83 R11.2
N$34
  Top 0.305: U$2.8 17.48,64.29 17.78,63.98 17.78,57.51 16.92,56.64 13.89,56.64 R13.1
N$35
  Top 0.406: U$3.3 U$3.4 U$3.5
  Top 1.778: U$3.4 38.79,15.16
  Top 1.93: U$6.P$2 30.48,11.4 | 30.48,11.4 35.03,11.4 38.79,15.16 | MAX_D.A 30.48,11.4
N$36  (via drill 0.6)
  Top 0.305: 18.12,28.93 U$1.4
  Top 0.61: 18.12,28.93 v15.24,28.93 14.73,28.93 13.08,30.58 C21.1
  Top 0.813: DSR2.1 15.52,39.83 v16.26,39.09
  Bottom 0.813: v16.26,39.09 15.24,38.07 v15.24,28.93
N$37  (via drill 0.6)
  Top 0.305: U$1.1 18.13,31.63 v17.78,31.98
  Top 0.406: C20.1 13.46,36.55 v17.78,36.55 24.89,36.55 25.91,35.53 25.91,30.45 25.04,29.59 U$1.6
  Bottom 0.305: v17.78,31.98 v17.78,36.55
N$38
  Top 0.406: U$3.10 40.7,21.93 | 42.24,20.4 MAX_R2.1 | MAX_R2.1 | U$3.16 36.89,21.5 37.08,21.31 | U$3.15 37.53,21.37 37.59,21.31
  Top 0.61: 37.08,21.31 37.47,21.31 37.53,21.37 | 37.59,21.31 40.64,21.31 | 40.64,21.31 41.33,21.31 42.24,20.4 | 40.7,21.93 40.7,21.37 40.64,21.31
  Top 1.422: MAX_R2.1 48.24,20.4 MAX_C5.1
N$39  (via drill 0.6)
  Top 0.305: v13.82,31.8 16.33,31.8 16.54,31.6 16.54,29.92 16.86,29.6 U$1.3 | v7.11,37.57 DSR3.1
  Bottom 0.305: v13.82,31.8 8.31,31.8 7.11,32.99 v7.11,37.57
N$40  (via drill 0.6)
  Top 0.406: U$3.8 41.34,19.6 40.64,20.29 36.07,20.29 v35.05,21.31 | v34.54,27.91 MAX_C4.2
  Bottom 0.406: v34.54,27.91 34.54,21.82 v35.05,21.31
N$41  (via drill 0.6)
  other vias: 6.88,65.25
N$42  (via drill 0.6)
  other vias: 17.02,65.28
N$43  (via drill 0.6)
  other vias: 18.52,65.3
N$44  (via drill 0.6)
  other vias: 19.68,64.64
N$45  (via drill 0.6)
  other vias: 20.73,63.53
N$51
  Top 0.406: U$2.10 U$2.9
  Top 0.61: C38.2 U$2.10
  Top 1.422: U$2.10 19.02,65.29 20.83,63.47 JP3.1 20.83,54.33
OSC1
  Top 0.305: C36.2 59.46,40.97 Q1.2 59.44,47.24 59.44,50.27 59.94,50.77 60.96,50.77 61.62,51.43 IC1.63
OSC2
  Top 0.305: C35.2 64.29,40.97 Q1.1 64.29,50.47 63.93,50.83 62.76,50.83 62.12,51.47 IC1.64
PGC2
  Top 0.305: IC1.26 38.27,69.12 38.02,69.37 J1.5
PGD2
  Top 0.305: IC1.27 37.02,68.62 36.07,69.57 36.07,71.09 36.58,71.6 37.26,71.6 37.69,72.03 38.25,72.03 J1.4
PIO  (via drill 0.6)
  Top 0.305: IC1.51 50.78,55.37 49.78,56.36 38.1,56.36 36.58,54.84 36.58,52.81 34.04,50.27 29.46,50.27 27.94,48.74 27.94,40.11 26.42,38.58 v24.38,38.58 | v23.88,35.03 23.88,31 U$1.8
  Bottom 0.305: v23.88,35.03 23.88,38.07 v24.38,38.58
REAL_BATT+
  Top 1.016: U$5.P1 7.12,42.71 DSR3.2 13.84,42.7 DSR2.2
  Top 1.422: U$5.P1 9.6,48.49 9.63,48.51
  Top 1.93: 20.02,48.51 20.78,48.51 JP1.3
  Top 2.184: 9.63,48.51 20.02,48.51
SCK1
  Top 0.305: IC1.55 57.62,53.43 56.52,52.32 49.28,52.32 48.54,51.59 48.54,51.54 47.75,50.75 47.75,49.25 47.24,48.74 JP7.3
SDI1
  Top 0.305: IC1.54 57.12,53.74 56.31,52.93 47.88,52.93 47.75,52.81 47.75,51.79 47.24,51.28 JP7.2
SDO1
  Top 0.305: IC1.53 56.62,54.05 56.16,53.59 47.98,53.59 47.75,53.82 JP7.1
VDD  (via drill 0.6, 1)
  Top 0.305: IC1.2 67.12,68.92 v66.75,68.55 67.06,68.25 67.06,62.97 67.9,62.12 IC1.86 | 51.41,62.23 C9.1 | IC1.16 60.12,69.75 v59.44,69.06 | IC1.30 56.05,67.12 v56.19,67.26 | IC1.46 55.16,59.12 v55.88,58.39 | v62.33,57.96 61.37,57.96 61.14,57.73 61.14,55.39 IC1.62 | IC1.37 52.8,63.62 51.41,62.23 | 51.41,62.23 51.41,61.04 v50.8,60.43
  Top 0.61: R4.2 56.01,81.13 v55.88,81.25
  Top 1.422: IC2.2 LMC2.1 35.03,60.96 v35.05,60.93
  Bottom 0.305: v66.75,68.55 65.68,68.55 65.08,67.94 C27.1 | v59.44,69.06 58.93,69.57 58.93,73.33 C5.1 | v56.19,67.26 C6.1 | v55.88,58.39 58.47,58.39 C13.1 | C16.1 62.35,57.99 v62.33,57.96 | v50.8,60.43 49.78,60.43
  Bottom 0.61: v55.88,81.25 55.37,81.25
  Bottom 0.813: C27.1 62.46,66.04 61.47,67.03 58.42,67.03
  Bottom 1.422: v35.05,60.93 36.58,60.93
  pour Bottom (isolate 0.254): 2.34,85.52 94.44,87.3 93.52,0.63 1.27,1.24 1.73,24.56
VDDUSB
  Top 0.406: U$2.1 U$2.2
  Top 0.61: JP4.VBUS1 6.1,65.28 | 6.1,65.28 6.41,65.28 6.43,65.3 | C37.2 10.8,67.85 10.34,67.39 U$2.1 | 6.1,65.28 6.1,69.06 5.59,69.57 3.48,69.57 2.69,70.36 2.69,74.23 LED3.A
  Top 1.27: LED1.A LED2.A LED3.A
  Top 1.422: U$2.1 6.44,65.29 6.43,65.3

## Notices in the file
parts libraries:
SparkFun-Retired: Licensing:Creative Commons ShareAlike 4.0 International - https://creativecommons.org/licenses/by-sa/4.0
